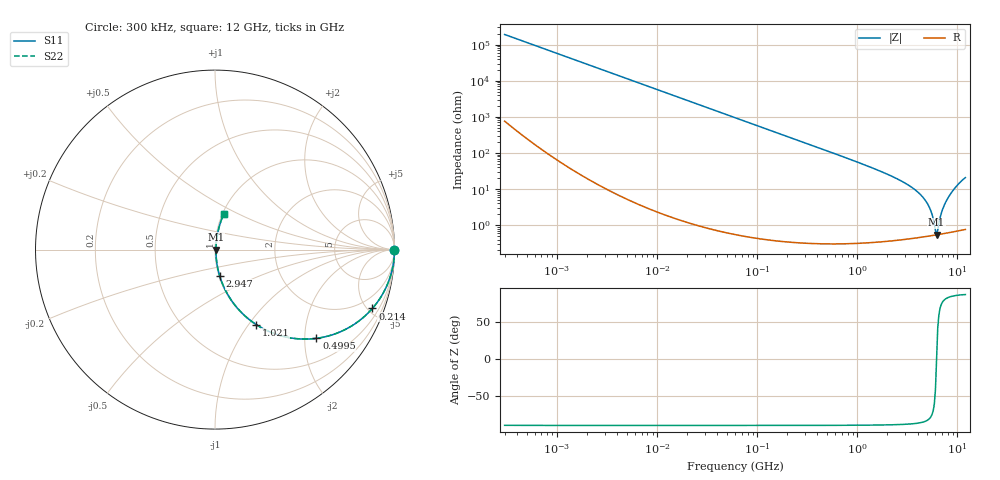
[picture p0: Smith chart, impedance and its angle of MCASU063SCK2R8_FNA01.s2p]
! MCASU063SCK2R8_FNA01  S-PARAMETER MODEL  ( General Type )
! Model Generated by TAIYO YUDEN Corporation (http://www.ty-top.com)
! Version 1.0
! TAIYO YUDEN Control No. 130801
! Copyright(c) 2013 TAIYO YUDEN CO.,LTD. All Rights Reserved.
! Product Description (link to TY-COMPAS)
! https://ds.yuden.co.jp/TYCOMPAS/or/detail?pn=MCASU063SCK2R8CFNA01&u=M
! Products Name : Multilayer Ceramic Capacitors
! Characteristics :
!  Capacitance : 2.8 pF , Rated Voltage : 50V , TCC : CK / C0K
!  Case Size : 0.6 x 0.3 / 0.024 x 0.012 [mm/inch] , Thickness : 0.3 / 0.012 [mm/inch]
!  (Conditions: Temperature = 25 degC , DC Bias Current/Voltage = 0A / 0V)
! External Node Assignments :
!  1  o---| |---o  2
! GND o---------o GND
! Frequency Range : 0.3MHz  -  12000MHz  [ 401 STEP ]
# MHz S RI R 50
! Freq[MHz].  S11 Real  S11 Imag  S21 Real  S21 Imag  S12 Real  S12 Imag  S22 Real  S22 Imag
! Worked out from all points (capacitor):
!   401 points, 300 kHz to 12 GHz, reference 50 ohm
!   read as one part in series: C = 2.78 pF near 316.3 kHz
!   lowest |Z| = 540 mohm at 6.188 GHz (marker M1)
!   series resonance near 6.181 GHz, so ESL is about 240 pH
!   S11 on the Smith chart (normalised r, x): 300 kHz: open; 214 MHz: 1.01, -5.35; 499.5 MHz: 1.01, -2.28; 1.021 GHz: 1.01, -1.09; 2.947 GHz: 1.01, -0.30; 12 GHz: 1.02, +0.41
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0.3  1 -0.000523  2.35e-06 0.000523  2.35e-06 0.000523  1 -0.000523
1.769972  1 -0.00309  1.18e-05 0.00309  1.18e-05 0.00309  1 -0.00309
10.44266  0.9997 -0.0182  0.000339 0.0182  0.000339 0.0182  0.9997 -0.0182
60  0.9891 -0.1035  0.0109 0.1035  0.0109 0.1035  0.9891 -0.1035
213.9924  0.8772 -0.3276  0.1228 0.3276  0.1228 0.3276  0.8772 -0.3276
353.9943  0.7224 -0.4469  0.2776 0.4469  0.2776 0.4469  0.7224 -0.4469
499.5319  0.5652 -0.4944  0.4348 0.4944  0.4348 0.4944  0.5652 -0.4944
1021.415  0.231 -0.4186  0.769 0.4186  0.769 0.4186  0.231 -0.4186
2088.533  0.0589 -0.2281  0.9411 0.2281  0.9411 0.2281  0.0589 -0.2281
2947.191  0.0258 -0.1459  0.9742 0.1459  0.9742 0.1459  0.0258 -0.1459
3944.255  0.0117 -0.0848  0.9883 0.0848  0.9883 0.0848  0.0117 -0.0848
4747.894  0.00719 -0.0489  0.9928 0.0489  0.9928 0.0489  0.00719 -0.0489
5278.635  0.00585 -0.0291  0.9942 0.0291  0.9942 0.0291  0.00585 -0.0291
5565.855  0.00549 -0.0193  0.9945 0.0193  0.9945 0.0193  0.00549 -0.0193
5868.704  0.00533 -0.00954  0.9947 0.00954  0.9947 0.00954  0.00533 -0.00954
6188.031  0.00537 0.000215  0.9946 -0.000215  0.9946 -0.000215  0.00537 0.000215
6524.734  0.00559 0.00965  0.9944 -0.00965  0.9944 -0.00965  0.00559 0.00965
6879.757  0.00603 0.0198  0.994 -0.0198  0.994 -0.0198  0.00603 0.0198
7254.098  0.00675 0.0309  0.9933 -0.0309  0.9933 -0.0309  0.00675 0.0309
8064.993  0.0093 0.0563  0.9907 -0.0563  0.9907 -0.0563  0.0093 0.0563
9968.853  0.0225 0.1239  0.9775 -0.1239  0.9775 -0.1239  0.0225 0.1239
12000  0.0478 0.1957  0.9522 -0.1957  0.9522 -0.1957  0.0478 0.1957
